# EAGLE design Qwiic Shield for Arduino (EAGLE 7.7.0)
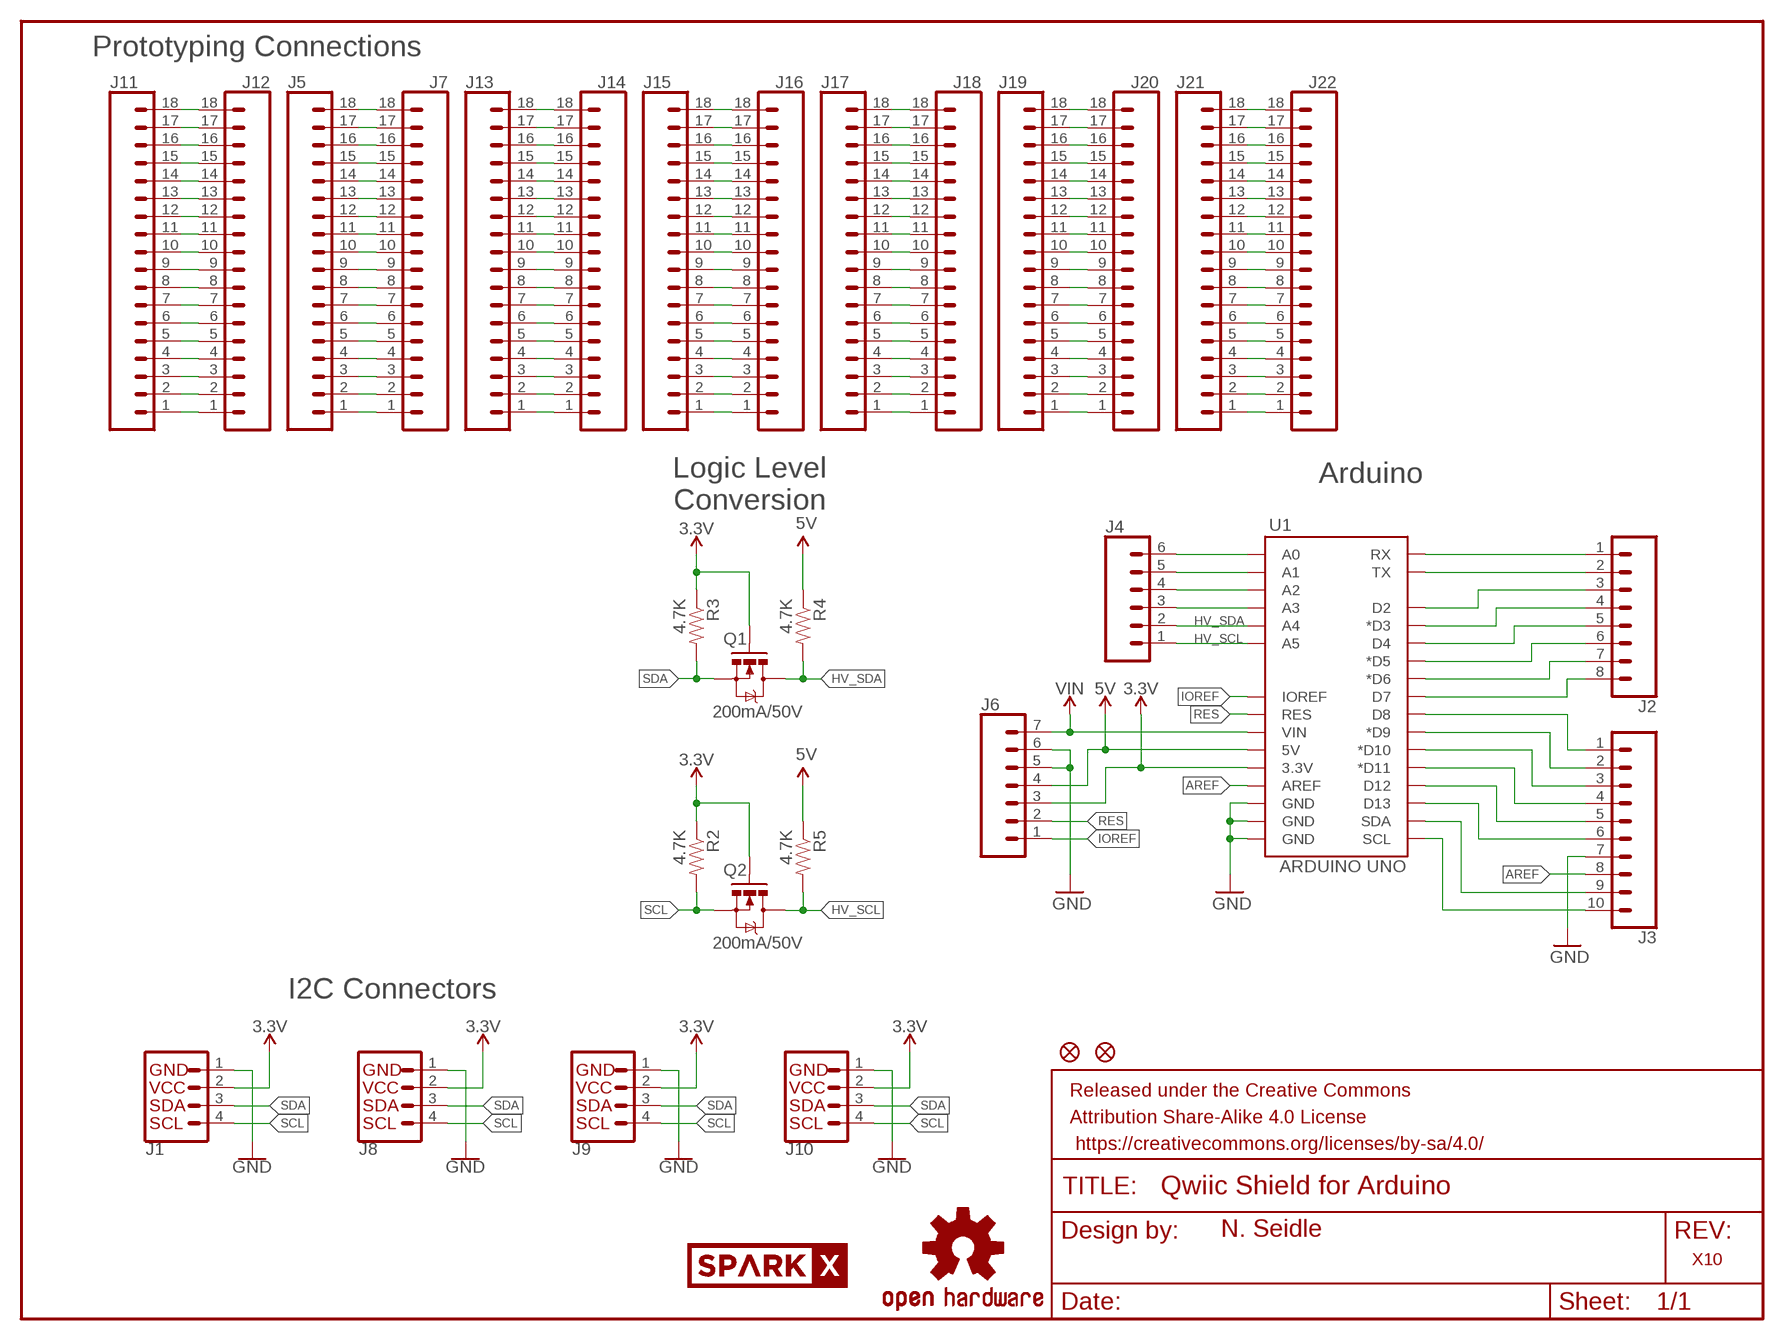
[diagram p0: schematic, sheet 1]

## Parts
FD1  FIDUCIAL1X2  [FIDUCIAL-1X2]
FD2  FIDUCIAL1X2  [FIDUCIAL-1X2]
FRAME1  FRAME-LETTER  [CREATIVE_COMMONS]
J1  I2C_STANDARDJS-1MM  [1X04_1MM_RA]
J2  CONN_08NO_SILK_FEMALE_PTH  [1X08_NO_SILK]
J3  CONN_10NO_SILK_PTH_FEMALE  [1X10_NO_SILK]
J4  CONN_06NO_SILK_FEMALE_PTH  [1X06_NO_SILK]
J5  CONN_18NO_SILK  [1X18_NO_SILK]
J6  CONN_07NO_SILK  [1X07_NO_SILK]
J7  CONN_18NO_SILK  [1X18_NO_SILK]
J8  I2C_STANDARDJS-1MM  [1X04_1MM_RA]
J9  I2C_STANDARDJS-1MM  [1X04_1MM_RA]
J10  I2C_STANDARDJS-1MM  [1X04_1MM_RA]
J11  CONN_18NO_SILK  [1X18_NO_SILK]
J12  CONN_18NO_SILK  [1X18_NO_SILK]
J13  CONN_18NO_SILK  [1X18_NO_SILK]
J14  CONN_18NO_SILK  [1X18_NO_SILK]
J15  CONN_18NO_SILK  [1X18_NO_SILK]
J16  CONN_18NO_SILK  [1X18_NO_SILK]
J17  CONN_18NO_SILK  [1X18_NO_SILK]
J18  CONN_18NO_SILK  [1X18_NO_SILK]
J19  CONN_18NO_SILK  [1X18_NO_SILK]
J20  CONN_18NO_SILK  [1X18_NO_SILK]
J21  CONN_18NO_SILK  [1X18_NO_SILK]
J22  CONN_18NO_SILK  [1X18_NO_SILK]
LOGO1  OSHW-LOGOMINI  [OSHW-LOGO-MINI]
Q1  200mA/50V  MOSFET-NCHANNELBSS138  [SOT23-3]
Q2  200mA/50V  MOSFET-NCHANNELBSS138  [SOT23-3]
R2  4.7K  4.7KOHM-1/10W-1%(0603)  [0603-RES]
R3  4.7K  4.7KOHM-1/10W-1%(0603)  [0603-RES]
R4  4.7K  4.7KOHM-1/10W-1%(0603)  [0603-RES]
R5  4.7K  4.7KOHM-1/10W-1%(0603)  [0603-RES]
U1  ARDUINO UNO  ARDUINO_R3_SHIELDNOLABELS  [UNO_R3_SHIELD_NOLABELS]
U$1  SPARKX-LOGO3  [SPARKX-SMALL]
U$2  SPARKX-LOGO5  [SPARKX-LARGE]

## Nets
3.3V: J1.2(VCC) J6.3 J8.2(VCC) J9.2(VCC) J10.2(VCC) Q1.1(G) Q2.1(G) R2.1 R3.1 U1.3.3V
5V: J6.4 R4.1 R5.1 U1.5V
A0: J4.6 U1.A0
A1: J4.5 U1.A1
A2: J4.4 U1.A2
A3: J4.3 U1.A3
AREF: J3.8 U1.AREF
D2: J2.3 U1.D2
D3: J2.4 U1.D3(*D3)
D4: J2.5 U1.D4
D5: J2.6 U1.D5(*D5)
D6: J2.7 U1.D6(*D6)
D7: J2.8 U1.D7
D8: J3.1 U1.D8
D9: J3.2 U1.D9(*D9)
D10: J3.3 U1.D10(*D10)
D11: J3.4 U1.D11(*D11)
D12: J3.5 U1.D12
D13: J3.6 U1.D13
GND [vcc]: J1.1(GND) J3.7 J6.5 J6.6 J8.1(GND) J9.1(GND) J10.1(GND) U1.GND@0(GND) U1.GND@1(GND) U1.GND@2(GND)
HV_SCL: J4.1 Q2.3(D) R5.2 U1.A5
HV_SDA: J4.2 Q1.3(D) R4.2 U1.A4
IOREF: J6.1 U1.IOREF
N$1: J5.2 J7.2
N$2: J5.3 J7.3
N$3: J5.4 J7.4
N$4: J5.5 J7.5
N$5: J5.6 J7.6
N$6: J5.7 J7.7
N$7: J5.8 J7.8
N$8: J5.9 J7.9
N$9: J5.10 J7.10
N$10: J5.11 J7.11
N$11: J5.12 J7.12
N$12: J5.13 J7.13
N$13: J5.14 J7.14
N$14: J5.15 J7.15
N$15: J5.16 J7.16
N$16: J5.17 J7.17
N$17: J5.18 J7.18
N$18: J5.1 J7.1
N$19: J13.2 J14.2
N$20: J13.3 J14.3
N$21: J11.2 J12.2
N$22: J11.3 J12.3
N$23: J11.4 J12.4
N$24: J11.5 J12.5
N$25: J11.6 J12.6
N$26: J11.7 J12.7
N$27: J11.8 J12.8
N$28: J11.9 J12.9
N$29: J11.10 J12.10
N$30: J11.11 J12.11
N$31: J11.12 J12.12
N$32: J11.13 J12.13
N$33: J11.14 J12.14
N$34: J11.15 J12.15
N$35: J11.16 J12.16
N$36: J11.17 J12.17
N$37: J11.18 J12.18
N$38: J11.1 J12.1
N$39: J13.4 J14.4
N$40: J13.5 J14.5
N$41: J13.6 J14.6
N$42: J13.7 J14.7
N$43: J13.8 J14.8
N$44: J13.9 J14.9
N$45: J13.10 J14.10
N$46: J13.11 J14.11
N$47: J13.12 J14.12
N$48: J13.13 J14.13
N$49: J13.14 J14.14
N$50: J13.15 J14.15
N$51: J13.16 J14.16
N$52: J13.17 J14.17
N$53: J13.18 J14.18
N$54: J13.1 J14.1
N$55: J15.2 J16.2
N$56: J15.3 J16.3
N$57: J15.4 J16.4
N$58: J15.5 J16.5
N$59: J15.6 J16.6
N$60: J15.7 J16.7
N$61: J15.8 J16.8
N$62: J15.9 J16.9
N$63: J15.10 J16.10
N$64: J15.11 J16.11
N$65: J15.12 J16.12
N$66: J15.13 J16.13
N$67: J15.14 J16.14
N$68: J15.15 J16.15
N$69: J15.16 J16.16
N$70: J15.17 J16.17
N$71: J15.18 J16.18
N$72: J15.1 J16.1
N$73: J17.2 J18.2
N$74: J17.3 J18.3
N$75: J17.4 J18.4
N$76: J17.5 J18.5
N$77: J17.6 J18.6
N$78: J17.7 J18.7
N$79: J17.8 J18.8
N$80: J17.9 J18.9
N$81: J17.10 J18.10
N$82: J17.11 J18.11
N$83: J17.12 J18.12
N$84: J17.13 J18.13
N$85: J17.14 J18.14
N$86: J17.15 J18.15
N$87: J17.16 J18.16
N$88: J17.17 J18.17
N$89: J17.18 J18.18
N$90: J17.1 J18.1
N$91: J19.2 J20.2
N$92: J19.3 J20.3
N$93: J19.4 J20.4
N$94: J19.5 J20.5
N$95: J19.6 J20.6
N$96: J19.7 J20.7
N$97: J19.8 J20.8
N$98: J19.9 J20.9
N$99: J19.10 J20.10
N$100: J19.11 J20.11
N$101: J19.12 J20.12
N$102: J19.13 J20.13
N$103: J19.14 J20.14
N$104: J19.15 J20.15
N$105: J19.16 J20.16
N$106: J19.17 J20.17
N$107: J19.18 J20.18
N$108: J19.1 J20.1
N$109: J21.2 J22.2
N$110: J21.3 J22.3
N$111: J21.4 J22.4
N$112: J21.5 J22.5
N$113: J21.6 J22.6
N$114: J21.7 J22.7
N$115: J21.8 J22.8
N$116: J21.9 J22.9
N$117: J21.10 J22.10
N$118: J21.11 J22.11
N$119: J21.12 J22.12
N$120: J21.13 J22.13
N$121: J21.14 J22.14
N$122: J21.15 J22.15
N$123: J21.16 J22.16
N$124: J21.17 J22.17
N$125: J21.18 J22.18
N$126: J21.1 J22.1
RES: J6.2 U1.RES
RX: J2.1 U1.RX
SCL: J1.4(SCL) J8.4(SCL) J9.4(SCL) J10.4(SCL) Q2.2(S) R2.2
SCL1: J3.10 U1.SCL
SDA: J1.3(SDA) J8.3(SDA) J9.3(SDA) J10.3(SDA) Q1.2(S) R3.2
SDA1: J3.9 U1.SDA
TX: J2.2 U1.TX
VIN [vcc]: J6.7 U1.VIN

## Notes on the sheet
- Prototyping Connections
- Logic Level
  Conversion
- Arduino
- I2C Connectors
- N. Seidle
- X10

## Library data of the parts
FD1 FD2 = SparkFun-Aesthetics:FIDUCIAL: Fiducial Alignment Points
FRAME1 = SparkFun-Aesthetics:FRAME-LETTER: Schematic Frame
J1 J8-J10 = SparkX:I2C_STANDARD: SparkFun I2C Standard Pinout Header SparkFun has standardized on a pinout for all I2C based sensor breakouts. This pinout allows I2C boards to be plugged directly into the headers on Arduino Uno compatible boards, and to be daisy chained easily. Example SparkFun Products: SparkFun Atmospheric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
J2 = SparkFun-Connectors:CONN_08: Multi connection point. Often used as Generic Header-pin footprint for 0.1 inch spaced/style header connections On any of the 0.1 inch spaced packages, you can populate with these: Break Away Headers - Straight (PRT-00116) Break Away Male Headers - Right Angle (PRT-00553) Female Headers (PRT-00115)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; PROD_ID: CONN-08438
J3 = SparkFun-Connectors:CONN_10: Multi connection point. Often used as Generic Header-pin footprint for 0.1 inch spaced/style header connections On any of the 0.1 inch spaced packages, you can populate with these: Break Away Headers - Straight (PRT-00116) Break Away Male Headers - Right Angle (PRT-00553) Female Headers (PRT-00115)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; PROD_ID: CONN-11563
J4 = SparkFun-Connectors:CONN_06: Multi connection point. Often used as Generic Header-pin footprint for 0.1 inch spaced/style header connections On any of the 0.1 inch spaced packages, you can populate with these: Break Away Headers - Straight (PRT-00116) Break Away Male Headers - Right Angle (PRT-00553) Female Headers (PRT-00115)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; PROD_ID: CONN-08437
J5 J7 J11-J22 = SparkX:CONN_18: Multi connection point. Often used as Generic Header-pin footprint for 0.1 inch spaced/style header connections On any of the 0.1 inch spaced packages, you can populate with these: Break Away Headers - Straight (PRT-00116) Break Away Male Headers - Right Angle (PRT-00553) Female Headers (PRT-00115)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
J6 = SparkFun-Connectors:CONN_07: Multi connection point. Often used as Generic Header-pin footprint for 0.1 inch spaced/style header connections On any of the 0.1 inch spaced packages, you can populate with these: Break Away Headers - Straight (PRT-00116) Break Away Male Headers - Right Angle (PRT-00553) Female Headers (PRT-00115)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
LOGO1 = SparkFun-Aesthetics:OSHW-LOGO: Open Source Hardware Logo
Q1 Q2 = SparkFun-DiscreteSemi:MOSFET-NCHANNEL: Common NMOSFET Parts MFG P/NStore IDProd ID FDD8780TRANS-09984 SI7820DNTRANS-11055 FDS6630AIC-08089 2N7002PWTRANS-11151 FQP30N06L COM-10213TRANS-10060 BSS123LT1GTRANS-08345 BSS138TRANS-00830 BS170 2N7000; PROD_ID: TRANS-00830
R2-R5 = SparkFun-Resistors:4.7KOHM-1/10W-1%(0603): RES-07857; PROD_ID: RES-07857
U1 = SparkFun-Boards:ARDUINO_R3_SHIELD: Shield form compatible with the Arduino Uno R3.
U$1 U$2 = SparkX:SPARKX-LOGO

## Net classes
0 Default: width 0.203 mm
1 vcc: width 0.203 mm

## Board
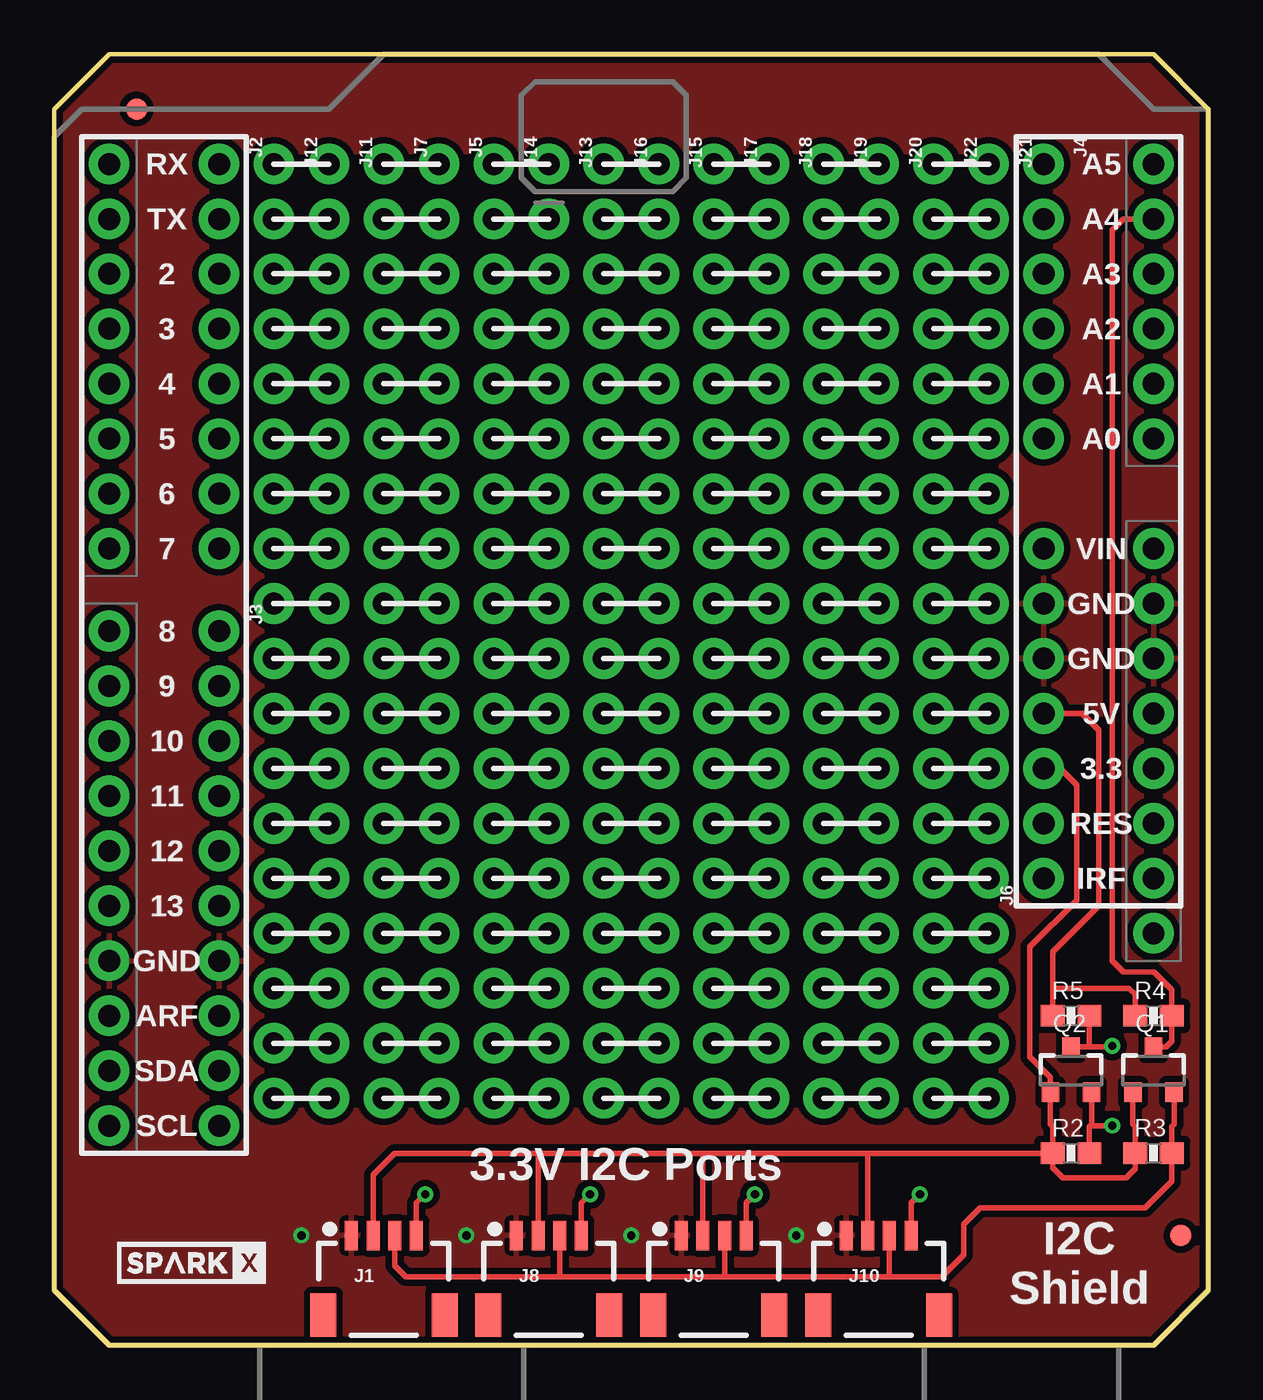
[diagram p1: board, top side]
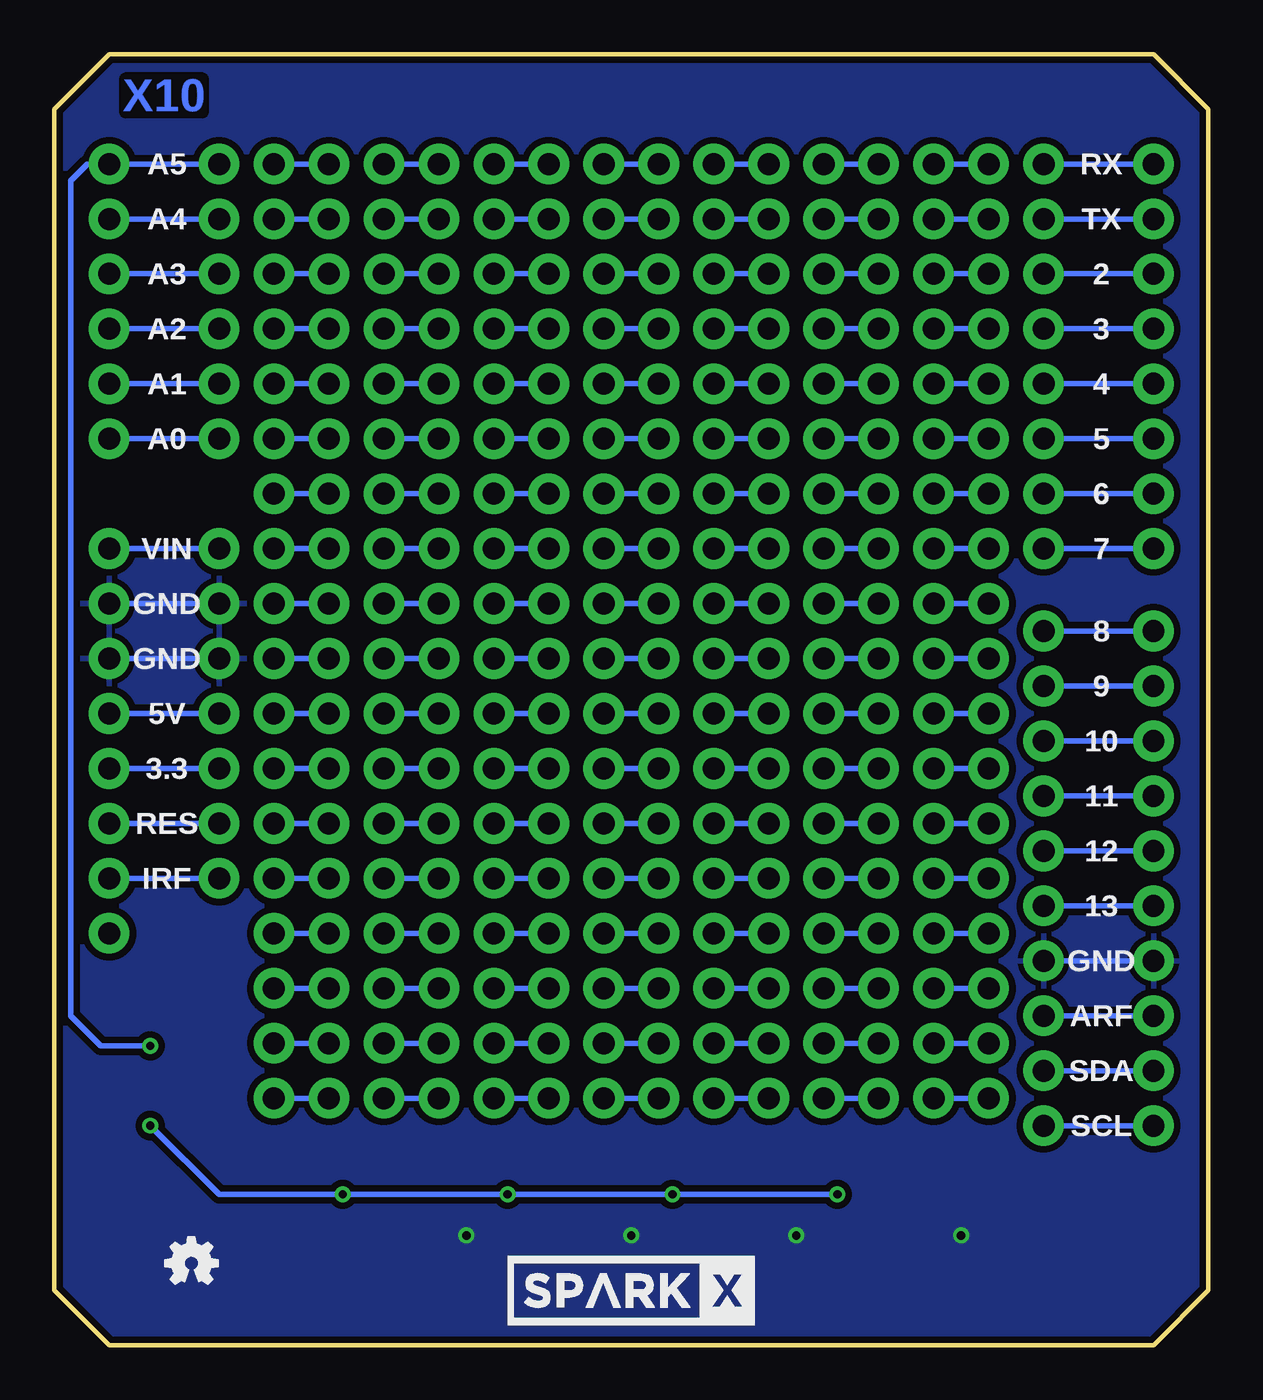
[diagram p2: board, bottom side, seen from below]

Size 53.34 x 59.69 mm. Coordinates in mm from the lower left corner, seen from the top.
Outline: 53.34,2.54 53.34,57.15 50.8,59.69 2.54,59.69 0,57.15 0,2.54 2.54,0 50.8,0 53.34,2.54
Copper layers (1*16): Top 0.035mm / dielectric 1.5mm / Bottom 0.035mm
Design rules "SparkFun-2-layer-TIGHT": minimum track width 7mil, minimum drill 15mil, track to track 7mil, track to pad 7mil, pad to pad 7mil, via to via 7mil, smd to smd 7mil, copper to edge 7mil, drill to drill 7mil, minimum pad ring 7mil, minimum via ring 7mil, stop-mask expansion 4mil, vias tented up to drill 25mil, thermal gap 10mil

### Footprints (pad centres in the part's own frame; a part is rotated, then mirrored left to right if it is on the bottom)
FIDUCIAL-1X2 = smd 1 x 1: 1 0,0
1X04_1MM_RA = smd 0.6 x 1.35: 1 -1.5,0; 2 -0.5,0; 3 0.5,0; 4 1.5,0 | smd 1.2 x 2: NC1 2.8,-3.675; NC2 -2.8,-3.675
1X08_NO_SILK = drill 1.016 pad 1.88: 1 0,0; 2 2.54,0; 3 5.08,0; 4 7.62,0; 5 10.16,0; 6 12.7,0; 7 15.24,0; 8 17.78,0
1X10_NO_SILK = drill 1.016 pad 1.88: 1 0,0; 2 2.54,0; 3 5.08,0; 4 7.62,0; 5 10.16,0; 6 12.7,0; 7 15.24,0; 8 17.78,0; 9 20.32,0; 10 22.86,0
1X06_NO_SILK = drill 1.016 pad 1.88: 1 0,0; 2 2.54,0; 3 5.08,0; 4 7.62,0; 5 10.16,0; 6 12.7,0
1X18_NO_SILK = drill 1.016 pad 1.88: 1 0,0; 2 2.54,0; 3 5.08,0; 4 7.62,0; 5 10.16,0; 6 12.7,0; 7 15.24,0; 8 17.78,0; 9 20.32,0; 10 22.86,0; 11 25.4,0; 12 27.94,0; 13 30.48,0; 14 33.02,0; 15 35.56,0; 16 38.1,0; 17 40.64,0; 18 43.18,0
1X07_NO_SILK = drill 1.016 pad 1.88: 1 0,0; 2 2.54,0; 3 5.08,0; 4 7.62,0; 5 10.16,0; 6 12.7,0; 7 15.24,0
SOT23-3 = smd 0.8 x 0.9: 1 -0.95,-1; 2 0.95,-1; 3 0,1.1
0603-RES = smd 1.1 x 1: 1 -0.85,0; 2 0.85,0
UNO_R3_SHIELD_NOLABELS = drill 1.016 pad 1.88: 3.3V 50.8,26.67; 5V 50.8,29.21; A0 50.8,41.91; A1 50.8,44.45; A2 50.8,46.99; A3 50.8,49.53; A4 50.8,52.07; A5 50.8,54.61; AREF 2.54,15.24; D2 2.54,49.53; D3 2.54,46.99; D4 2.54,44.45; D5 2.54,41.91; D6 2.54,39.37; D7 2.54,36.83; D8 2.54,33.02; D9 2.54,30.48; D10 2.54,27.94; D11 2.54,25.4; D12 2.54,22.86; D13 2.54,20.32; GND@0 50.8,31.75; GND@1 50.8,34.29; GND@2 2.54,17.78; IOREF 50.8,21.59; NC 50.8,19.05; RES 50.8,24.13; RX 2.54,54.61; SCL 2.54,10.16; SDA 2.54,12.7; TX 2.54,52.07; VIN 50.8,36.83

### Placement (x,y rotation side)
FD1  52.07,5.08 0 top
FD2  3.81,57.15 0 top
FRAME1  not placed on the board
J1  15.24,5.08 0 top
J2  7.62,54.61 270 top
J3  7.62,33.02 270 top
J4  45.72,54.61 270 top
J5  17.78,54.61 270 top
J6  45.72,21.59 90 top
J7  15.24,54.61 270 top
J8  22.86,5.08 0 top
J9  30.48,5.08 0 top
J10  38.1,5.08 0 top
J11  12.7,54.61 270 top
J12  10.16,54.61 270 top
J13  22.86,54.61 270 top
J14  20.32,54.61 270 top
J15  27.94,54.61 270 top
J16  25.4,54.61 270 top
J17  30.48,54.61 270 top
J18  33.02,54.61 270 top
J19  35.56,54.61 270 top
J20  38.1,54.61 270 top
J21  43.18,54.61 270 top
J22  40.64,54.61 270 top
LOGO1  46.99,3.81 0 bottom
Q1  50.8,12.7 0 top
Q2  46.99,12.7 0 top
R2  46.99,8.89 0 top
R3  50.8,8.89 0 top
R4  50.8,15.24 0 top
R5  46.99,15.24 0 top
U1  0,0 0 top
U$1  6.35,3.81 0 top
U$2  26.67,2.54 0 bottom

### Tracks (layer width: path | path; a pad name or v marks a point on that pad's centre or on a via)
3.3V
  Top 0.254: R2.1 37.59,8.89 | 37.59,8.89 29.97,8.89 | 29.97,8.89 22.35,8.89 | 22.35,8.89 15.75,8.89 14.74,7.88 J1.2 | J8.2 22.36,8.88 22.35,8.89 | J9.2 29.98,8.88 29.97,8.89 | J10.2 37.6,8.88 37.59,8.89 | R2.1 46.14,10.12 46.04,10.22 Q2.1 46.04,12.38 45.09,13.34 45.09,18.41 47.24,20.57 47.24,25.91 46.48,26.67 J6.3 | Q1.1 49.85,10.22 49.95,10.12 R3.1 49.95,8.17 49.53,7.75 46.61,7.75 46.14,8.22 R2.1
  Bottom 0.254: J6.3 U1.3.3V
5V
  Top 0.254: R4.1 49.95,16.22 49.66,16.51 46.14,16.51 | R5.1 46.14,16.51 | 46.14,16.51 46.14,18.2 48.26,20.32 48.26,28.45 47.5,29.21 J6.4
  Bottom 0.254: J6.4 U1.5V
A0
  Bottom 0.254: J4.6 U1.A0
A1
  Bottom 0.254: U1.A1 J4.5
A2
  Bottom 0.254: J4.4 U1.A2
A3
  Bottom 0.254: U1.A3 J4.3
AREF
  Bottom 0.254: U1.AREF J3.8
D2
  Bottom 0.254: J2.3 U1.D2
D3
  Bottom 0.254: U1.D3 J2.4
D4
  Bottom 0.254: J2.5 U1.D4
D5
  Bottom 0.254: U1.D5 J2.6
D6
  Bottom 0.254: J2.7 U1.D6
D7
  Bottom 0.254: U1.D7 J2.8
D8
  Bottom 0.254: J3.1 U1.D8
D9
  Bottom 0.254: U1.D9 J3.2
D10
  Bottom 0.254: J3.3 U1.D10
D11
  Bottom 0.254: U1.D11 J3.4
D12
  Bottom 0.254: J3.5 U1.D12
D13
  Bottom 0.254: U1.D13 J3.6
GND  (via drill 0.38)
  Bottom 0.254: U1.GND@1 J6.6 | J6.5 U1.GND@0 | J3.7 U1.GND@2
  other vias: 34.29,5.08 26.67,5.08 19.05,5.08 11.43,5.08
  pour Top (isolate 0.305): 53.34,0 0,0 0,59.69 53.34,59.69
  pour Bottom (isolate 0.305): 53.34,0 0,0 0,59.69 53.34,59.69
HV_SCL  (via drill 0.38)
  Top 0.254: Q2.3 47.88,13.8 | 47.88,13.8 48.85,13.8 v48.9,13.84 | R5.2 47.84,13.84 47.88,13.8
  Bottom 0.254: J4.1 U1.A5 51.82,54.61 52.58,53.85 52.58,15.24 51.18,13.84 v48.9,13.84
HV_SDA
  Top 0.254: Q1.3 51.39,13.8 51.65,14.06 R4.2 51.65,16.42 50.8,17.27 49.4,17.27 48.9,17.78 48.9,51.56 49.4,52.07 U1.A4
  Bottom 0.254: J4.2 U1.A4
IOREF
  Bottom 0.254: J6.1 U1.IOREF
N$1
  Bottom 0.254: J7.2 J5.2
N$2
  Bottom 0.254: J5.3 J7.3
N$3
  Bottom 0.254: J7.4 J5.4
N$4
  Bottom 0.254: J5.5 J7.5
N$5
  Bottom 0.254: J7.6 J5.6
N$6
  Bottom 0.254: J5.7 J7.7
N$7
  Bottom 0.254: J7.8 J5.8
N$8
  Bottom 0.254: J5.9 J7.9
N$9
  Bottom 0.254: J7.10 J5.10
N$10
  Bottom 0.254: J5.11 J7.11
N$11
  Bottom 0.254: J7.12 J5.12
N$12
  Bottom 0.254: J5.13 J7.13
N$13
  Bottom 0.254: J7.14 J5.14
N$14
  Bottom 0.254: J5.15 J7.15
N$15
  Bottom 0.254: J7.16 J5.16
N$16
  Bottom 0.254: J5.17 J7.17
N$17
  Bottom 0.254: J7.18 J5.18
N$18
  Bottom 0.254: J5.1 J7.1
N$19
  Bottom 0.254: J14.2 J13.2
N$20
  Bottom 0.254: J13.3 J14.3
N$21
  Bottom 0.254: J11.2 J12.2
N$22
  Bottom 0.254: J12.3 J11.3
N$23
  Bottom 0.254: J11.4 J12.4
N$24
  Bottom 0.254: J12.5 J11.5
N$25
  Bottom 0.254: J12.6 J11.6
N$26
  Bottom 0.254: J11.7 J12.7
N$27
  Bottom 0.254: J12.8 J11.8
N$28
  Bottom 0.254: J11.9 J12.9
N$29
  Bottom 0.254: J12.10 J11.10
N$30
  Bottom 0.254: J11.11 J12.11
N$31
  Bottom 0.254: J12.12 J11.12
N$32
  Bottom 0.254: J11.13 J12.13
N$33
  Bottom 0.254: J12.14 J11.14
N$34
  Bottom 0.254: J11.15 J12.15
N$35
  Bottom 0.254: J12.16 J11.16
N$36
  Bottom 0.254: J11.17 J12.17
N$37
  Bottom 0.254: J12.18 J11.18
N$38
  Bottom 0.254: J12.1 J11.1
N$39
  Bottom 0.254: J14.4 J13.4
N$40
  Bottom 0.254: J13.5 J14.5
N$41
  Bottom 0.254: J14.6 J13.6
N$42
  Bottom 0.254: J13.7 J14.7
N$43
  Bottom 0.254: J14.8 J13.8
N$44
  Bottom 0.254: J13.9 J14.9
N$45
  Bottom 0.254: J14.10 J13.10
N$46
  Bottom 0.254: J13.11 J14.11
N$47
  Bottom 0.254: J14.12 J13.12
N$48
  Bottom 0.254: J13.13 J14.13
N$49
  Bottom 0.254: J14.14 J13.14
N$50
  Bottom 0.254: J13.15 J14.15
N$51
  Bottom 0.254: J14.16 J13.16
N$52
  Bottom 0.254: J13.17 J14.17
N$53
  Bottom 0.254: J14.18 J13.18
N$54
  Bottom 0.254: J13.1 J14.1
N$55
  Bottom 0.254: J16.2 J15.2
N$56
  Bottom 0.254: J15.3 J16.3
N$57
  Bottom 0.254: J15.4 J16.4
N$58
  Bottom 0.254: J16.5 J15.5
N$59
  Bottom 0.254: J15.6 J16.6
N$60
  Bottom 0.254: J16.7 J15.7
N$61
  Bottom 0.254: J15.8 J16.8
N$62
  Bottom 0.254: J16.9 J15.9
N$63
  Bottom 0.254: J16.10 J15.10
N$64
  Bottom 0.254: J15.11 J16.11
N$65
  Bottom 0.254: J16.12 J15.12
N$66
  Bottom 0.254: J15.13 J16.13
N$67
  Bottom 0.254: J16.14 J15.14
N$68
  Bottom 0.254: J15.15 J16.15
N$69
  Bottom 0.254: J16.16 J15.16
N$70
  Bottom 0.254: J15.17 J16.17
N$71
  Bottom 0.254: J16.18 J15.18
N$72
  Bottom 0.254: J15.1 J16.1
N$73
  Bottom 0.254: J17.2 J18.2
N$74
  Bottom 0.254: J18.3 J17.3
N$75
  Bottom 0.254: J17.4 J18.4
N$76
  Bottom 0.254: J18.5 J17.5
N$77
  Bottom 0.254: J17.6 J18.6
N$78
  Bottom 0.254: J18.7 J17.7
N$79
  Bottom 0.254: J17.8 J18.8
N$80
  Bottom 0.254: J18.9 J17.9
N$81
  Bottom 0.254: J18.10 J17.10
N$82
  Bottom 0.254: J17.11 J18.11
N$83
  Bottom 0.254: J18.12 J17.12
N$84
  Bottom 0.254: J17.13 J18.13
N$85
  Bottom 0.254: J18.14 J17.14
N$86
  Bottom 0.254: J18.15 J17.15
N$87
  Bottom 0.254: J17.16 J18.16
N$88
  Bottom 0.254: J18.17 J17.17
N$89
  Bottom 0.254: J17.18 J18.18
N$90
  Bottom 0.254: J18.1 J17.1
N$91
  Bottom 0.254: J19.2 J20.2
N$92
  Bottom 0.254: J20.3 J19.3
N$93
  Bottom 0.254: J20.4 J19.4
N$94
  Bottom 0.254: J19.5 J20.5
N$95
  Bottom 0.254: J20.6 J19.6
N$96
  Bottom 0.254: J19.7 J20.7
N$97
  Bottom 0.254: J20.8 J19.8
N$98
  Bottom 0.254: J19.9 J20.9
N$99
  Bottom 0.254: J19.10 J20.10
N$100
  Bottom 0.254: J20.11 J19.11
N$101
  Bottom 0.254: J19.12 J20.12
N$102
  Bottom 0.254: J20.13 J19.13
N$103
  Bottom 0.254: J19.14 J20.14
N$104
  Bottom 0.254: J20.15 J19.15
N$105
  Bottom 0.254: J19.16 J20.16
N$106
  Bottom 0.254: J20.17 J19.17
N$107
  Bottom 0.254: J19.18 J20.18
N$108
  Bottom 0.254: J20.1 J19.1
N$109
  Bottom 0.254: J21.2 J22.2
N$110
  Bottom 0.254: J22.3 J21.3
N$111
  Bottom 0.254: J21.4 J22.4
N$112
  Bottom 0.254: J22.5 J21.5
N$113
  Bottom 0.254: J21.6 J22.6
N$114
  Bottom 0.254: J22.7 J21.7
N$115
  Bottom 0.254: J21.8 J22.8
N$116
  Bottom 0.254: J22.9 J21.9
N$117
  Bottom 0.254: J22.10 J21.10
N$118
  Bottom 0.254: J21.11 J22.11
N$119
  Bottom 0.254: J22.12 J21.12
N$120
  Bottom 0.254: J21.13 J22.13
N$121
  Bottom 0.254: J22.14 J21.14
N$122
  Bottom 0.254: J21.15 J22.15
N$123
  Bottom 0.254: J22.16 J21.16
N$124
  Bottom 0.254: J21.17 J22.17
N$125
  Bottom 0.254: J22.18 J21.18
N$126
  Bottom 0.254: J22.1 J21.1
RES
  Bottom 0.254: U1.RES J6.2
RX
  Bottom 0.254: J2.1 U1.RX
SCL  (via drill 0.38)
  Top 0.254: Q2.2 47.94,10.22 | 47.94,10.22 47.84,10.12 R2.2 | J10.4 39.6,6.58 v40.01,6.99 | v48.9,10.16 48,10.16 47.94,10.22 | J9.4 31.98,6.58 v32.38,6.99 | J8.4 24.36,6.58 v24.77,6.99 | J1.4 16.74,6.58 v17.14,6.99
  Bottom 0.254: v48.9,10.16 45.72,6.99 v40.01,6.99 v32.38,6.99 v24.77,6.99 v17.14,6.99
SCL1
  Bottom 0.254: J3.10 U1.SCL
SDA
  Top 0.254: Q1.2 51.75,10.22 51.65,10.12 R3.2 51.65,7.58 50.42,6.35 42.8,6.35 42.04,5.59 42.04,4.19 41.02,3.17 38.61,3.17 | J1.3 15.74,3.69 16.26,3.17 23.37,3.17 | 23.37,3.17 30.99,3.17 | 30.99,3.17 38.61,3.17 | J10.3 38.6,3.18 38.61,3.17 | J9.3 30.98,3.18 30.99,3.17 | J8.3 23.36,3.18 23.37,3.17
SDA1
  Bottom 0.254: U1.SDA J3.9
TX
  Bottom 0.254: U1.TX J2.2
VIN
  Bottom 0.254: J6.7 U1.VIN

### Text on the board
Bottom: X10
tPlace: RX | A5 | TX | A4 | 2 | A3 | 3 | A2 | 4 | A1 | 5 | A0 | 6 | 7 | VIN | GND | 8 | GND | 9 | 5V | 10 | 3.3 | 11 | RES | 12 | IRF | 13 | GND | ARF | SDA | SCL | 3.3V I2C Ports | I2C / Shield
bPlace: RX | A5 | TX | A4 | 2 | A3 | 3 | A2 | 4 | A1 | 5 | A0 | 6 | 7 | VIN | GND | 8 | GND | 9 | 5V | 10 | 3.3 | 11 | RES | 12 | IRF | 13 | GND | ARF | SDA | SCL
tDocu: N. Seidle

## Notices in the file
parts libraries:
SparkFun-Boards: Licensing: CC v3.0 Share-Alike You are welcome to use this library for commercial purposes.
SparkFun-Aesthetics: Released under the Creative Commons Attribution Share-Alike 4.0 License
SparkFun-Aesthetics: https://creativecommons.org/licenses/by-sa/4.0
